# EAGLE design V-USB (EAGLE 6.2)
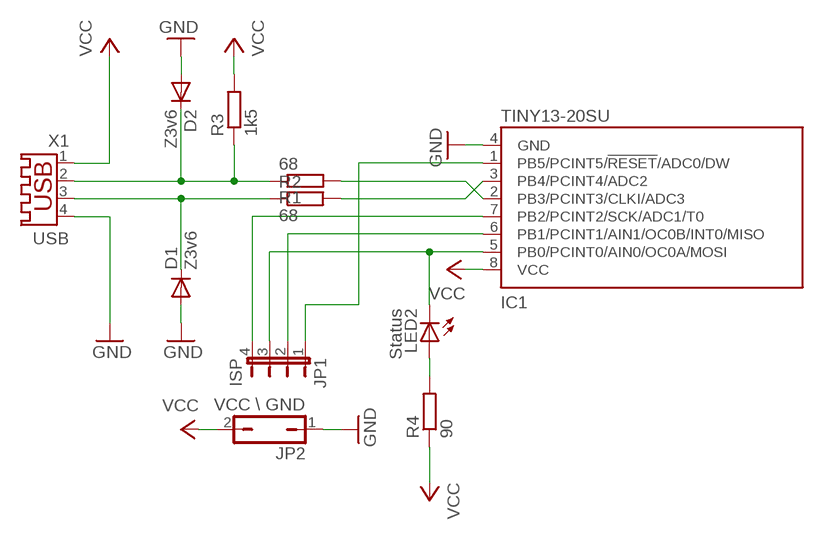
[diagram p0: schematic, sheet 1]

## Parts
D1  Z3v6  DIODE-MINIMELF  [MINIMELF]
D2  Z3v6  DIODE-MINIMELF  [MINIMELF]
IC1  TINY13-20SU  [8S2]
JP1  ISP  JP4E  [JP4]
JP2  VCC \ GND  JP1Q  [JP1]
LED2  Status  LEDCHIPLED_1206  [CHIPLED_1206]
R1  68  R-EU_M0805  [M0805]
R2  68  R-EU_M0805  [M0805]
R3  1k5  R-EU_M0805  [M0805]
R4  90  R-EU_M0805  [M0805]
X1  USB  USB-A003  [USB-A003]

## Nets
GND: D1.A D2.A IC1.4(GND) JP2.1 X1.4
N$1: D1.C R2.1 X1.3
N$2: D2.C R1.1 R3.1 X1.2
N$3: IC1.3(PB4/PCINT4/ADC2) R2.2
N$4: IC1.2(PB3/PCINT3/CLKI/ADC3) R1.2
N$5: IC1.5(PB0/PCINT0/AIN0/OC0A/MOSI) JP1.3 LED2.C
N$7: IC1.7(PB2/PCINT2/SCK/ADC1/T0) JP1.4
N$8: IC1.1(PB5/PCINT5/!RESET!/ADC0/DW) JP1.1
N$9: LED2.A R4.2
N$10: IC1.6(PB1/PCINT1/AIN1/OC0B/INT0/MISO) JP1.2
VCC: IC1.8(VCC) JP2.2 R3.2 R4.1 X1.1

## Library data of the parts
D1 D2 = diode:DIODE-: DIODE
IC1 = atmel:TINY13: 8-bit AVR Microcontroller with 1K Bytes In-System Programmable Flash Source: http://www.atmel.com/dyn/resources/prod_documents/2535S.pdf; MPN: ATTINY13-20SU; OC_FARNELL: 9171568; OC_NEWARK: 96K6522
JP1 = jumper:JP4E: JUMPER
JP2 = jumper:JP1Q: JUMPER
LED2 = led:LED: LED
R1-R4 = rcl:R-EU_: RESISTOR, European symbol
X1 = con-yamaichi:USB-A003: USB connector; OC_FARNELL: unknown; OC_NEWARK: unknown

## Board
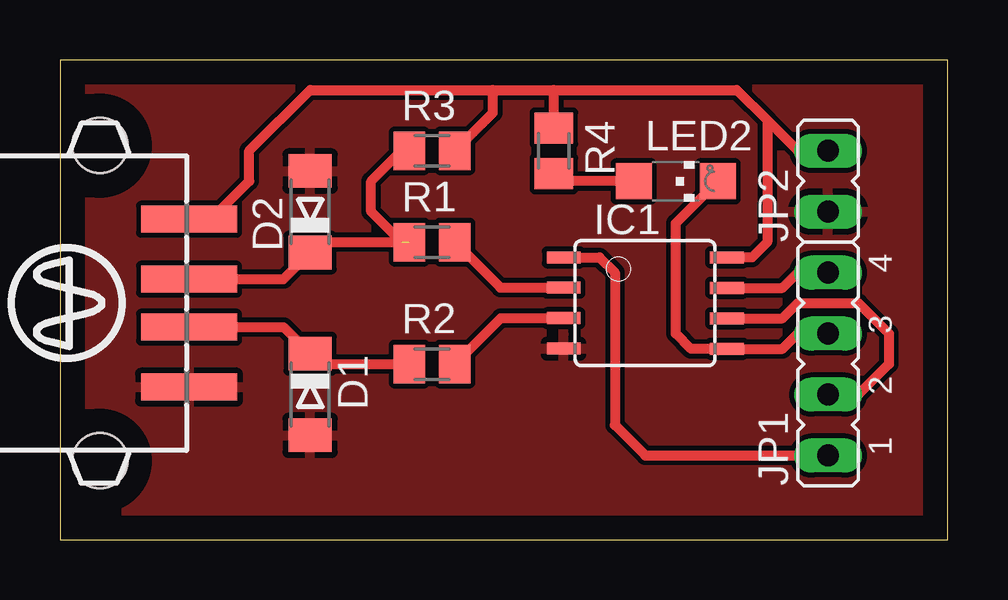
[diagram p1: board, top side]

Size 37 x 20 mm. Coordinates in mm from the lower left corner, seen from the top.
Outline: 0,0 37,0 37,20 0,20 0,0
Copper layers (1*16): Top 0.035mm / dielectric 1.5mm / Bottom 0.035mm
Design rules: minimum track width 10mil, minimum drill 24mil, track to track 8mil, track to pad 8mil, pad to pad 8mil, via to via 8mil, smd to smd 8mil, copper to edge 40mil, drill to drill 8mil, minimum pad ring 10mil, minimum via ring 8mil, stop-mask expansion 4mil, vias tented up to drill 0mil, thermal gap 10mil

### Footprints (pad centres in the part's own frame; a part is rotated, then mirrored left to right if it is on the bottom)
MINIMELF = smd 1.4 x 1.8: A 1.7,0; C -1.7,0
8S2 = smd 0.5 x 1.4: 1 -1.905,-3.404; 2 -0.645,-3.404; 3 0.625,-3.404; 4 1.895,-3.404; 5 1.905,3.404; 6 0.635,3.404; 7 -0.635,3.404; 8 -1.905,3.404
JP4 = drill 0.914 long: 1 -3.81,0; 2 -1.27,0; 3 1.27,0; 4 3.81,0
JP1 = drill 0.914 long: 1 0,-1.27; 2 0,1.27
CHIPLED_1206 = smd 1.5 x 1.5: A 0,-1.75; C 0,1.75
M0805 = smd 1.3 x 1.6: 1 -0.95,0; 2 0.95,0
USB-A003 = smd 1.12 x 4: 1 -3.5,14; 2 -1,14; 3 1,14; 4 3.5,14 | hole 2.3: -6.57,10.28; 6.57,10.28

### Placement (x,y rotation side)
D1  10.43,6.05 270 top
D2  10.43,13.67 90 top
IC1  24.4,9.86 270 top
JP1  32.02,7.32 90 top
JP2  32.02,14.94 0 top
LED2  25.67,14.94 270 top
R1  15.51,12.4 0 top
R2  15.51,7.32 0 top
R3  15.51,16.21 0 top
R4  20.59,16.21 270 top
X1  -8.62,9.86 270 top

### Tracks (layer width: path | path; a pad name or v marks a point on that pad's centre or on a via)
GND
  pour Top: 37,0 0,0 0,20 37,20
N$1
  Top 0.406: X1.3 9.32,8.86 D1.C 10.86,7.32 R2.1
N$2  (1 unrouted)
  Top 0.406: X1.2 9.32,10.86 D2.C 10.86,12.4 14.24,12.4 12.97,13.67 12.97,14.94 14.24,16.21 R3.1
N$3
  Top 0.406: R2.2 18.38,9.23 IC1.3
N$4
  Top 0.406: R1.2 18.36,10.5 IC1.2
N$5
  Top 0.406: LED2.C 25.67,13.19 25.67,8.59 26.3,7.95 IC1.5 30.11,7.95 30.75,8.59 JP1.3
N$7
  Top 0.406: IC1.7 30.11,10.5 30.75,11.13 JP1.4
N$8
  Top 0.406: IC1.1 22.5,11.77 23.13,11.13 23.13,4.78 24.4,3.51 JP1.1
N$9
  Top 0.406: LED2.A 20.91,14.94 R4.2
N$10
  Top 0.406: IC1.6 30.11,9.23 30.75,9.86 33.29,9.86 34.56,8.59 34.56,7.32 33.29,6.05 JP1.2
VCC
  Top 0.406: X1.1 6.31,13.36 7.89,14.94 7.89,16.21 10.43,18.75 18.05,18.75 | 18.05,18.75 20.59,18.75 | 20.59,18.75 28.21,18.75 29.48,17.48 | 18.05,18.75 18.05,17.8 R3.2 | IC1.8 28.84,11.77 29.48,12.4 29.48,17.48 | R4.1 20.59,18.75 | JP2.2 30.75,16.21 29.48,17.48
